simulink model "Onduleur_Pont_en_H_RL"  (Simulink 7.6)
settings: Solver=ode15s  StartTime=0.0  StopTime=10  RelTol=1e-3
InitFcn:
  | clc
  | R=1e3; C=2500e-3/(5*pi);%1e-3/(5*pi)
  | 
  | R1=1e3
  | R2=R1;
StopFcn:
  | if 0
  | clc
  | close all, clc
  | load U_Umoy_charge.mat
  | plot(x(1,:),x(2,:),x(1,:),x(3,:))
  | xlabel('temps')
  | title('Tension charge et sa valeur moyenne')
  | grid
  | 
  | load I_Imoy_charge.mat
  | figure
  | plot(y(1,:),y(2,:),y(1,:),y(3,:))
  | xlabel('temps')
  | title('Courant charge et sa valeur moyenne')
  | grid
  | 
  | delete *.mat
  | end
libraries: fl_lib x33, nesl_utility x16, powerlib x10, elec_lib x6

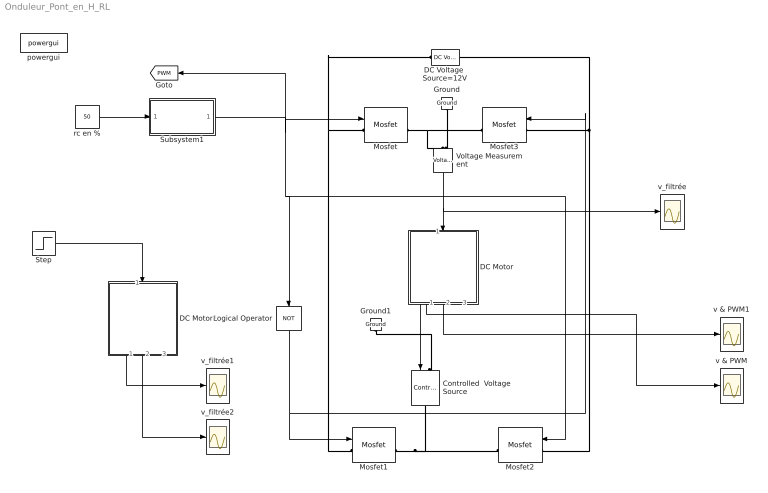
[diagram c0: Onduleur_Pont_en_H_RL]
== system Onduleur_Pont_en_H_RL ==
  Controlled  Voltage Source : powerlib/Electrical Sources/Controlled Voltage Source  DialogController=POWERSYS.PowerSysDialog  SystemSampleTime=-1  Initialize=on  Source_Type=AC  Amplitude=0  Phase=0  Frequency=0  Measurements=None
  DC Motor : Subsystem
  DC Motor1 : Subsystem
  DC Voltage  Source=12V : powerlib/Electrical Sources/DC Voltage Source  DialogController=POWERSYS.PowerSysDialog  SystemSampleTime=-1  Amplitude=12  Measurements=None
  Ground : powerlib/Elements/Ground  DialogController=POWERSYS.PowerSysDialog  PhysicalDomain=powersysdomain  SubClassName=unknown  LeftPortType=p1  RightPortType=p1  LConnTagsString=a
  Ground1 : powerlib/Elements/Ground  DialogController=POWERSYS.PowerSysDialog  PhysicalDomain=powersysdomain  SubClassName=unknown  LeftPortType=p1  RightPortType=p1  LConnTagsString=a
  Logical Operator : Logic  Operator=NOT  AllPortsSameDT=off  OutDataTypeStr=boolean
  Mosfet{,1..3} (4 alike) : powerlib/Power Electronics/Mosfet  DialogController=POWERSYS.PowerSysDialog  SystemSampleTime=-1  Ron=1e-6  Lon=0  Rd=0.001  Vfd=0  IC=0  Rs=1e8  Cs=inf  Measurements=on
  Step : Step  Time=2  After=12  SampleTime=0
  Subsystem1 : Subsystem
  Voltage Measurement : powerlib/Measurements/Voltage Measurement  DialogController=POWERSYS.PowerSysDialog  SystemSampleTime=-1  PhasorSimulation=off  OutputType=Complex  PSBequivalent=0
  powergui : powerlib/powergui  SystemSampleTime=-1  SimulationMode=Continuous  SampleTime=0  frequency=60  SPID=off  DisableSnubberDevices=off  DisableRonSwitches=off  DisableVfSwitches=off  SwTol=0  Interpol=off  frequencyindice=0  echomessages=off  HookPort=off  DisplayEquations=off  FunctionMessages=off  EnableUseOfTLC=off  x0status=blocks  RestoreLinks=warning  ResistiveCurrentMeasurement=off  Frange=[0:2:500]  Ylog=off  Xlog=on  ShowGrid=off  save=off  variable=ZData  ZoomFFT=on  StartTime=0.0  cycles=1  DisplayStyle=1  fundamental=60  FreqAxis=off  MaxFrequency=1000  frequencyindicesteady=1  RmsSteady=1  display=off  Ts=0  methode=off
  rc en % : Constant  Value=50
  v & PWM : Scope
  v & PWM1 : Scope
  v_filtrée : Scope
  v_filtrée1 : Scope
  v_filtrée2 : Scope
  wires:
  Subsystem1/1(PWM) -> Mosfet/1, Logical Operator/1, Mosfet2/1, [PWM]
  rc en %/1 -> Subsystem1/1(rc (%))
  Logical Operator/1 -> Mosfet1/1, Mosfet3/1
  Voltage Measurement/1 -> DC Motor/1(U+), v_filtrée/1
  DC Motor/3(U-) -> Controlled  Voltage Source/1
  DC Motor/1(w) -> v & PWM/1
  DC Motor/2(alpha) -> v & PWM1/1
  Step/1 -> DC Motor1/1(U+)
  DC Motor1/1(w) -> v_filtrée1/1
  DC Motor1/2(alpha) -> v_filtrée2/1
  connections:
  Mosfet1/RConn1 -- Mosfet2/RConn1 -- Controlled  Voltage Source/RConn1
  Mosfet/RConn1 -- Mosfet3/RConn1 -- Voltage Measurement/LConn1
  Mosfet1/LConn1 -- DC Voltage  Source=12V/LConn1 -- Mosfet/LConn1
  Mosfet2/LConn1 -- Mosfet3/LConn1 -- DC Voltage  Source=12V/RConn1
  Ground/LConn1 -- Voltage Measurement/LConn2
  Ground1/LConn1 -- Controlled  Voltage Source/LConn1

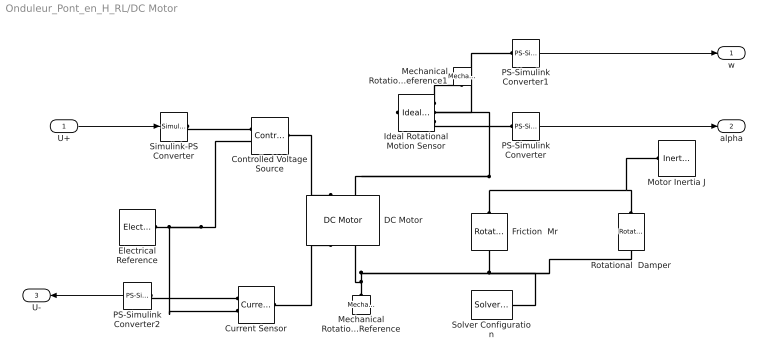
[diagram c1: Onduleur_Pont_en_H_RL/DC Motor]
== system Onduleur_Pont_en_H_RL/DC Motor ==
  U+ : Inport
  Controlled Voltage Source : fl_lib/Electrical/Electrical Sources/Controlled Voltage Source  DialogController=NetworkEngine.DynNeDlgSource  SystemSampleTime=-1  i_Log=off  v_Log=off  LocalVarNames=|i|v  LocalVarDescs=|i|v  LocalVarLogging=[0 0]
  Current Sensor : fl_lib/Electrical/Electrical Sensors/Current Sensor  DialogController=NetworkEngine.DynNeDlgSource  SystemSampleTime=-1  i1_Log=off  v1_Log=off  LocalVarNames=|i1|v1  LocalVarDescs=|i1|v1  LocalVarLogging=[0 0]
  DC Motor : elec_lib/Actuators & Drivers/Rotational Actuators/DC Motor  DialogController=NetworkEngine.DynNeDlgSource  SystemSampleTime=-1  parameterization=1  Ra=3.9 Ohm  La=1.2e-3 H  emf_or_torque=2  Kv=7.2e-5 V/rpm  Ki=10e-3 N*m/A  T_stall=2.4e-4 N*m  w_max=1.91e+4 rpm  w_rated=1.5e+4 rpm  P_rated=0.08 W  V_rated=1.5 V  J=0.01 g*cm^2  lam=1e-8 N*m/(rad/s)  speed0=0 rpm  current_Log=off  voltage_Log=off  power_Log=off  i2r_Log=off  torque_Log=off  speed_Log=off  LocalVarNames=|current|voltage|power|i2r|torque|speed  LocalVarDescs=|Current (A)|Voltage (V)|Power (W)|Electrical losses (W)|Torque (Nm)|Angular speed (rad/s)  LocalVarLogging=[0 0 0 0 0 0]
  Electrical Reference : fl_lib/Electrical/Electrical Elements/Electrical Reference  DialogController=NetworkEngine.DynNeDlgSource  SystemSampleTime=-1  i_Log=off  LocalVarNames=|i  LocalVarDescs=|i  LocalVarLogging=0
  Friction  Mr : fl_lib/Mechanical/Rotational Elements/Rotational Friction  DialogController=NetworkEngine.DynNeDlgSource  SystemSampleTime=-1  brkwy_trq=0.01e-3 N*m  Col_trq=0.01e-3 N*m  visc_coef=0.001e-3 N*m/(rad/s)  trans_coef=10 s/rad  vel_thr=0.1 rad/s  t_Log=off  w_Log=off  LocalVarNames=|friction_torque|rel_velocity|power  LocalVarDescs=|Friction torque (N*m)|Relative velocity (rad/s)|Power (W)  LocalVarLogging=[0 0 0]
  Ideal Rotational Motion Sensor : fl_lib/Mechanical/Mechanical Sensors/Ideal Rotational Motion Sensor  DialogController=NetworkEngine.DynNeDlgSource  SystemSampleTime=-1  offset=0 rad  w_Log=off  t_Log=off  phi_Log=off  LocalVarNames=|w|t|phi  LocalVarDescs=|w|t|phi  LocalVarLogging=[0 0 0]
  Mechanical Rotational Reference : fl_lib/Mechanical/Rotational Elements/Mechanical Rotational Reference  DialogController=NetworkEngine.DynNeDlgSource  SystemSampleTime=-1  t_Log=off  LocalVarNames=|t  LocalVarDescs=|t  LocalVarLogging=0
  Mechanical Rotational Reference1 : fl_lib/Mechanical/Rotational Elements/Mechanical Rotational Reference  DialogController=NetworkEngine.DynNeDlgSource  SystemSampleTime=-1  t_Log=off  LocalVarNames=|t  LocalVarDescs=|t  LocalVarLogging=0
  Motor Inertia J : fl_lib/Mechanical/Rotational Elements/Inertia  DialogController=NetworkEngine.DynNeDlgSource  SystemSampleTime=-1  inertia=0.01 g*cm^2  initial_velocity=0 rad/s  t_Log=off  LocalVarNames=|torque|velocity  LocalVarDescs=|Inertia torque (N*m)|Inertia absolute velocity (rad/s)  LocalVarLogging=[0 0]
  PS-Simulink Converter : nesl_utility/PS-Simulink Converter  DialogController=NetworkEngine.DynNeUtilDlgSource  SystemSampleTime=-1  PhysicalDomain=network_engine_domain  LeftPortType=input  RightPortType=output  SubClassName=ps_output  Unit=1  AffineConversion=off
  PS-Simulink Converter1 : nesl_utility/PS-Simulink Converter  DialogController=NetworkEngine.DynNeUtilDlgSource  SystemSampleTime=-1  PhysicalDomain=network_engine_domain  LeftPortType=input  RightPortType=output  SubClassName=ps_output  Unit=1  AffineConversion=off
  PS-Simulink Converter2 : nesl_utility/PS-Simulink Converter  DialogController=NetworkEngine.DynNeUtilDlgSource  SystemSampleTime=-1  PhysicalDomain=network_engine_domain  LeftPortType=input  RightPortType=output  SubClassName=ps_output  Unit=1  AffineConversion=off
  Rotational  Damper : fl_lib/Mechanical/Rotational Elements/Rotational Damper  DialogController=NetworkEngine.DynNeDlgSource  SystemSampleTime=-1  D=0.01 N*m/(rad/s)  t_Log=off  w_Log=off  LocalVarNames=|t|w  LocalVarDescs=|t|w  LocalVarLogging=[0 0]
  Simulink-PS Converter : nesl_utility/Simulink-PS Converter  DialogController=NetworkEngine.DynNeUtilDlgSource  SystemSampleTime=-1  PhysicalDomain=network_engine_domain  LeftPortType=input  RightPortType=output  SubClassName=ps_input  Unit=1  AffineConversion=off  InputFilterTimeConstant=.001  UdotUserProvided=0
  Solver Configuration : nesl_utility/Solver Configuration  DialogController=NetworkEngine.DynNeUtilDlgSource  SystemSampleTime=-1  PhysicalDomain=network_engine_domain  LeftPortType=input  RightPortType=generic  SubClassName=solver  Accelerate=off  Profile=off  ResidualTolerance=1e-9  MaxNonlinIter=3  MaxModeIter=2  DoFixedCost=off  UseLocalSampling=off  DoDC=off  LinearAlgebra=Sparse  LocalSolverSampleTime=.001  LocalSolverChoice=NE_BACKWARD_EULER_ADVANCER  UseLocalSolver=off
  w : Outport
  alpha : Outport  Port=2
  U- : Outport  Port=3
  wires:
  PS-Simulink Converter2/1 -> U-/1
  PS-Simulink Converter1/1 -> w/1
  PS-Simulink Converter/1 -> alpha/1
  U+/1 -> Simulink-PS Converter/1
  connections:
  PS-Simulink Converter2/LConn1 -- Current Sensor/RConn1
  Electrical Reference/LConn1 -- Current Sensor/RConn2 -- Controlled Voltage Source/RConn2
  Ideal Rotational Motion Sensor/RConn3 -- PS-Simulink Converter/LConn1
  Ideal Rotational Motion Sensor/RConn2 -- PS-Simulink Converter1/LConn1
  Ideal Rotational Motion Sensor/RConn1 -- Mechanical Rotational Reference1/LConn1
  Mechanical Rotational Reference/LConn1 -- DC Motor/RConn2 -- Friction  Mr/RConn1 -- Rotational  Damper/RConn1 -- Solver Configuration/RConn1
  Rotational  Damper/LConn1 -- Ideal Rotational Motion Sensor/LConn1 -- DC Motor/LConn2 -- Friction  Mr/LConn1 -- Motor Inertia J/LConn1
  Current Sensor/LConn1 -- DC Motor/RConn1
  Simulink-PS Converter/RConn1 -- Controlled Voltage Source/RConn1
  Controlled Voltage Source/LConn1 -- DC Motor/LConn1

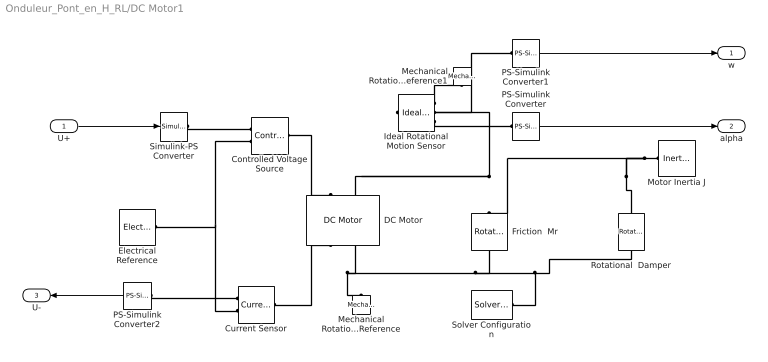
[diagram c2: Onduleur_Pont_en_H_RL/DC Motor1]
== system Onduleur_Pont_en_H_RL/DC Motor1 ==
  U+ : Inport
  Controlled Voltage Source : fl_lib/Electrical/Electrical Sources/Controlled Voltage Source  DialogController=NetworkEngine.DynNeDlgSource  SystemSampleTime=-1  i_Log=off  v_Log=off  LocalVarNames=|i|v  LocalVarDescs=|i|v  LocalVarLogging=[0 0]
  Current Sensor : fl_lib/Electrical/Electrical Sensors/Current Sensor  DialogController=NetworkEngine.DynNeDlgSource  SystemSampleTime=-1  i1_Log=off  v1_Log=off  LocalVarNames=|i1|v1  LocalVarDescs=|i1|v1  LocalVarLogging=[0 0]
  DC Motor : elec_lib/Actuators & Drivers/Rotational Actuators/DC Motor  DialogController=NetworkEngine.DynNeDlgSource  SystemSampleTime=-1  parameterization=1  Ra=3.9 Ohm  La=1.2e-3 H  emf_or_torque=2  Kv=7.2e-5 V/rpm  Ki=10e-3 N*m/A  T_stall=2.4e-4 N*m  w_max=1.91e+4 rpm  w_rated=1.5e+4 rpm  P_rated=0.08 W  V_rated=1.5 V  J=0.01 g*cm^2  lam=1e-8 N*m/(rad/s)  speed0=0 rpm  current_Log=off  voltage_Log=off  power_Log=off  i2r_Log=off  torque_Log=off  speed_Log=off  LocalVarNames=|current|voltage|power|i2r|torque|speed  LocalVarDescs=|Current (A)|Voltage (V)|Power (W)|Electrical losses (W)|Torque (Nm)|Angular speed (rad/s)  LocalVarLogging=[0 0 0 0 0 0]
  Electrical Reference : fl_lib/Electrical/Electrical Elements/Electrical Reference  DialogController=NetworkEngine.DynNeDlgSource  SystemSampleTime=-1  i_Log=off  LocalVarNames=|i  LocalVarDescs=|i  LocalVarLogging=0
  Friction  Mr : fl_lib/Mechanical/Rotational Elements/Rotational Friction  DialogController=NetworkEngine.DynNeDlgSource  SystemSampleTime=-1  brkwy_trq=0.001 N*m  Col_trq=0.001 N*m  visc_coef=0.001 N*m/(rad/s)  trans_coef=10 s/rad  vel_thr=0.1 rad/s  t_Log=off  w_Log=off  LocalVarNames=|friction_torque|rel_velocity|power  LocalVarDescs=|Friction torque (N*m)|Relative velocity (rad/s)|Power (W)  LocalVarLogging=[0 0 0]
  Ideal Rotational Motion Sensor : fl_lib/Mechanical/Mechanical Sensors/Ideal Rotational Motion Sensor  DialogController=NetworkEngine.DynNeDlgSource  SystemSampleTime=-1  offset=0 rad  w_Log=off  t_Log=off  phi_Log=off  LocalVarNames=|w|t|phi  LocalVarDescs=|w|t|phi  LocalVarLogging=[0 0 0]
  Mechanical Rotational Reference : fl_lib/Mechanical/Rotational Elements/Mechanical Rotational Reference  DialogController=NetworkEngine.DynNeDlgSource  SystemSampleTime=-1  t_Log=off  LocalVarNames=|t  LocalVarDescs=|t  LocalVarLogging=0
  Mechanical Rotational Reference1 : fl_lib/Mechanical/Rotational Elements/Mechanical Rotational Reference  DialogController=NetworkEngine.DynNeDlgSource  SystemSampleTime=-1  t_Log=off  LocalVarNames=|t  LocalVarDescs=|t  LocalVarLogging=0
  Motor Inertia J : fl_lib/Mechanical/Rotational Elements/Inertia  DialogController=NetworkEngine.DynNeDlgSource  SystemSampleTime=-1  inertia=0.1 g*cm^2  initial_velocity=0 rad/s  t_Log=off  LocalVarNames=|torque|velocity  LocalVarDescs=|Inertia torque (N*m)|Inertia absolute velocity (rad/s)  LocalVarLogging=[0 0]
  PS-Simulink Converter : nesl_utility/PS-Simulink Converter  DialogController=NetworkEngine.DynNeUtilDlgSource  SystemSampleTime=-1  PhysicalDomain=network_engine_domain  LeftPortType=input  RightPortType=output  SubClassName=ps_output  Unit=1  AffineConversion=off
  PS-Simulink Converter1 : nesl_utility/PS-Simulink Converter  DialogController=NetworkEngine.DynNeUtilDlgSource  SystemSampleTime=-1  PhysicalDomain=network_engine_domain  LeftPortType=input  RightPortType=output  SubClassName=ps_output  Unit=1  AffineConversion=off
  PS-Simulink Converter2 : nesl_utility/PS-Simulink Converter  DialogController=NetworkEngine.DynNeUtilDlgSource  SystemSampleTime=-1  PhysicalDomain=network_engine_domain  LeftPortType=input  RightPortType=output  SubClassName=ps_output  Unit=1  AffineConversion=off
  Rotational  Damper : fl_lib/Mechanical/Rotational Elements/Rotational Damper  DialogController=NetworkEngine.DynNeDlgSource  SystemSampleTime=-1  D=0.01 N*m/(rad/s)  t_Log=off  w_Log=off  LocalVarNames=|t|w  LocalVarDescs=|t|w  LocalVarLogging=[0 0]
  Simulink-PS Converter : nesl_utility/Simulink-PS Converter  DialogController=NetworkEngine.DynNeUtilDlgSource  SystemSampleTime=-1  PhysicalDomain=network_engine_domain  LeftPortType=input  RightPortType=output  SubClassName=ps_input  Unit=1  AffineConversion=off  InputFilterTimeConstant=.001  UdotUserProvided=0
  Solver Configuration : nesl_utility/Solver Configuration  DialogController=NetworkEngine.DynNeUtilDlgSource  SystemSampleTime=-1  PhysicalDomain=network_engine_domain  LeftPortType=input  RightPortType=generic  SubClassName=solver  Accelerate=off  Profile=off  ResidualTolerance=1e-9  MaxNonlinIter=3  MaxModeIter=2  DoFixedCost=off  UseLocalSampling=off  DoDC=off  LinearAlgebra=Sparse  LocalSolverSampleTime=.001  LocalSolverChoice=NE_BACKWARD_EULER_ADVANCER  UseLocalSolver=off
  w : Outport
  alpha : Outport  Port=2
  U- : Outport  Port=3
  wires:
  U+/1 -> Simulink-PS Converter/1
  PS-Simulink Converter/1 -> alpha/1
  PS-Simulink Converter1/1 -> w/1
  PS-Simulink Converter2/1 -> U-/1
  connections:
  Controlled Voltage Source/LConn1 -- DC Motor/LConn1
  Simulink-PS Converter/RConn1 -- Controlled Voltage Source/RConn1
  Current Sensor/LConn1 -- DC Motor/RConn1
  Motor Inertia J/LConn1 -- Friction  Mr/LConn1 -- DC Motor/LConn2 -- Ideal Rotational Motion Sensor/LConn1 -- Rotational  Damper/LConn1
  Solver Configuration/RConn1 -- Rotational  Damper/RConn1 -- Friction  Mr/RConn1 -- DC Motor/RConn2 -- Mechanical Rotational Reference/LConn1
  Ideal Rotational Motion Sensor/RConn1 -- Mechanical Rotational Reference1/LConn1
  Ideal Rotational Motion Sensor/RConn2 -- PS-Simulink Converter1/LConn1
  Ideal Rotational Motion Sensor/RConn3 -- PS-Simulink Converter/LConn1
  Controlled Voltage Source/RConn2 -- Current Sensor/RConn2 -- Electrical Reference/LConn1
  PS-Simulink Converter2/LConn1 -- Current Sensor/RConn1

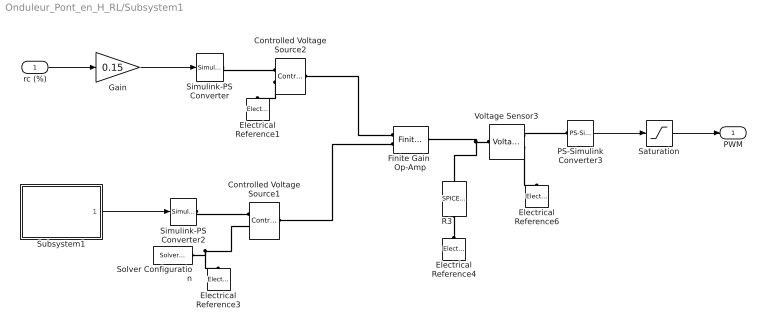
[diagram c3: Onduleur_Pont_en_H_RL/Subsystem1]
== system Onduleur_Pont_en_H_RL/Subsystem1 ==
  rc (%) : Inport
  Controlled Voltage Source1 : fl_lib/Electrical/Electrical Sources/Controlled Voltage Source  DialogController=NetworkEngine.DynNeDlgSource  SystemSampleTime=-1  i_Log=off  v_Log=off  LocalVarNames=|current|voltage|power  LocalVarDescs=|Current (A)|Voltage (V)|Power (W)  LocalVarLogging=[0 0 0]
  Controlled Voltage Source2 : fl_lib/Electrical/Electrical Sources/Controlled Voltage Source  DialogController=NetworkEngine.DynNeDlgSource  SystemSampleTime=-1  i_Log=off  v_Log=off  LocalVarNames=|current|voltage|power  LocalVarDescs=|Current (A)|Voltage (V)|Power (W)  LocalVarLogging=[0 0 0]
  Electrical Reference{1,3..4,6} (4 alike) : fl_lib/Electrical/Electrical Elements/Electrical Reference  DialogController=NetworkEngine.DynNeDlgSource  SystemSampleTime=-1  i_Log=off  LocalVarNames=|i  LocalVarDescs=|i  LocalVarLogging=[]
  Finite Gain  Op-Amp : elec_lib/Integrated Circuits/Finite Gain Op-Amp  DialogController=NetworkEngine.DynNeDlgSource  SystemSampleTime=-1  A=1000  Rin=1e+06 Ohm  Rout=100 Ohm  Vmin=-12 V  Vmax=12 V  LocalVarNames=|power  LocalVarDescs=|Dissipated power (W)  LocalVarLogging=0
  Gain : Gain  Gain=0.15
  PS-Simulink Converter3 : nesl_utility/PS-Simulink Converter  DialogController=NetworkEngine.DynNeUtilDlgSource  SystemSampleTime=-1  PhysicalDomain=network_engine_domain  LeftPortType=input  RightPortType=output  SubClassName=ps_output  Unit=1  AffineConversion=off
  R3 : elec_lib/Additional Components/SPICE-Compatible Components/Passive Devices/SPICE Resistor  DialogController=NetworkEngine.DynNeDlgSource  SystemSampleTime=-1  SCALE=1  R_param=1  R=10e3 Ohm  RSH=0 Ohm  LENGTH=1e-06 m  WIDTH=1e-06 m  NARROW=0 m  T_param=1  TC1=0 1/K  TC2=0 1/K^2  TOFFSET=0 K  TFIXED=300.15 K  TMEAS=300.15 K  LocalVarLogging=[]
  Saturation : Saturate  UpperLimit=1  LowerLimit=0
  Simulink-PS Converter : nesl_utility/Simulink-PS Converter  DialogController=NetworkEngine.DynNeUtilDlgSource  SystemSampleTime=-1  PhysicalDomain=network_engine_domain  LeftPortType=input  RightPortType=output  SubClassName=ps_input  Unit=1  AffineConversion=off  InputFilterTimeConstant=.001  UdotUserProvided=0
  Simulink-PS Converter2 : nesl_utility/Simulink-PS Converter  DialogController=NetworkEngine.DynNeUtilDlgSource  SystemSampleTime=-1  PhysicalDomain=network_engine_domain  LeftPortType=input  RightPortType=output  SubClassName=ps_input  Unit=1  AffineConversion=off  InputFilterTimeConstant=.001  UdotUserProvided=0
  Solver Configuration : nesl_utility/Solver Configuration  DialogController=NetworkEngine.DynNeUtilDlgSource  SystemSampleTime=-1  PhysicalDomain=network_engine_domain  LeftPortType=input  RightPortType=generic  SubClassName=solver  Accelerate=off  Profile=off  ResidualTolerance=1e-12  MaxNonlinIter=12  MaxModeIter=2  DoFixedCost=on  UseLocalSampling=off  DoDC=off  LinearAlgebra=Sparse  LocalSolverSampleTime=.001  LocalSolverChoice=NE_BACKWARD_EULER_ADVANCER  UseLocalSolver=off
  Subsystem1 : Subsystem
  Voltage Sensor3 : fl_lib/Electrical/Electrical Sensors/Voltage Sensor  DialogController=NetworkEngine.DynNeDlgSource  SystemSampleTime=-1  i1_Log=off  v1_Log=off  LocalVarNames=|i1|v1  LocalVarDescs=|i1|v1  LocalVarLogging=[]
  PWM : Outport
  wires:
  Gain/1 -> Simulink-PS Converter/1
  Saturation/1 -> PWM/1
  PS-Simulink Converter3/1 -> Saturation/1
  rc (%)/1 -> Gain/1
  Subsystem1/1(tri) -> Simulink-PS Converter2/1
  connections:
  Voltage Sensor3/RConn1 -- PS-Simulink Converter3/LConn1
  Voltage Sensor3/LConn1 -- R3/RConn1 -- Finite Gain  Op-Amp/RConn1
  Voltage Sensor3/RConn2 -- Electrical Reference6/LConn1
  Electrical Reference4/LConn1 -- R3/LConn1
  Controlled Voltage Source2/RConn2 -- Electrical Reference1/LConn1
  Simulink-PS Converter/RConn1 -- Controlled Voltage Source2/RConn1
  Finite Gain  Op-Amp/LConn1 -- Controlled Voltage Source2/LConn1
  Solver Configuration/RConn1 -- Electrical Reference3/LConn1 -- Controlled Voltage Source1/RConn2
  Simulink-PS Converter2/RConn1 -- Controlled Voltage Source1/RConn1
  Controlled Voltage Source1/LConn1 -- Finite Gain  Op-Amp/LConn2

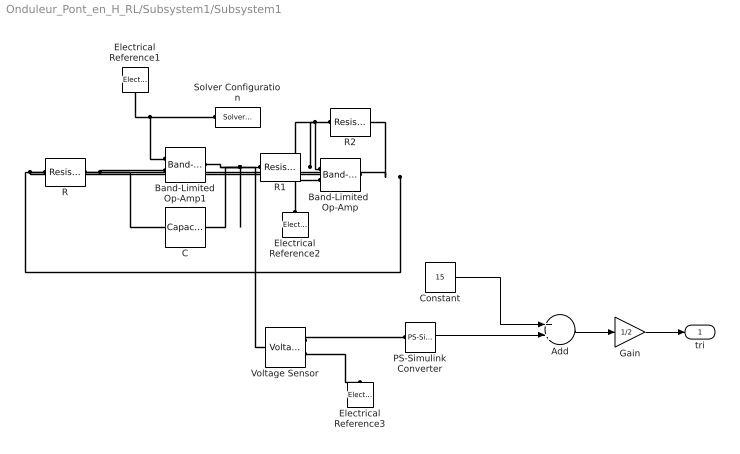
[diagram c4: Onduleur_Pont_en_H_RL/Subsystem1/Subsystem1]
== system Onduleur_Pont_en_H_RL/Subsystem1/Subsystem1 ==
  Add : Sum
  Band-Limited  Op-Amp : elec_lib/Integrated Circuits/Band-Limited Op-Amp  DialogController=NetworkEngine.DynNeDlgSource  SystemSampleTime=-1  A=1000  Rin=1e+06 Ohm  Rout=100 Ohm  Vmin=-15 V  Vmax=15 V  Vdotmax=1000 V/s  f=1e+05 Hz  V0=0 V  LocalVarNames=|power  LocalVarDescs=|Dissipated power (W)  LocalVarLogging=0
  Band-Limited Op-Amp1 : elec_lib/Integrated Circuits/Band-Limited Op-Amp  DialogController=NetworkEngine.DynNeDlgSource  SystemSampleTime=-1  A=1000  Rin=1e+06 Ohm  Rout=100 Ohm  Vmin=-15 V  Vmax=15 V  Vdotmax=1000 V/s  f=1e+05 Hz  V0=0 V  LocalVarNames=|power  LocalVarDescs=|Dissipated power (W)  LocalVarLogging=0
  C : fl_lib/Electrical/Electrical Elements/Capacitor  DialogController=NetworkEngine.DynNeDlgSource  SystemSampleTime=-1  c=0.5e-4 F  v0=0.1 V  r=1e-6 Ohm  g=0 1/Ohm  i_Log=off  v_Log=off  vc_Log=off  LocalVarNames=|current|voltage|power  LocalVarDescs=|Capacitor current (A)|Voltage across capacitor (V)|Power (W)  LocalVarLogging=[0 0 0]
  Constant : Constant  Value=15
  Electrical Reference1 : fl_lib/Electrical/Electrical Elements/Electrical Reference  DialogController=NetworkEngine.DynNeDlgSource  SystemSampleTime=-1  i_Log=off  LocalVarNames=|i  LocalVarDescs=|i  LocalVarLogging=[]
  Electrical Reference2 : fl_lib/Electrical/Electrical Elements/Electrical Reference  DialogController=NetworkEngine.DynNeDlgSource  SystemSampleTime=-1  i_Log=off  LocalVarNames=|i  LocalVarDescs=|i  LocalVarLogging=[]
  Electrical Reference3 : fl_lib/Electrical/Electrical Elements/Electrical Reference  DialogController=NetworkEngine.DynNeDlgSource  SystemSampleTime=-1  i_Log=off  LocalVarNames=|i  LocalVarDescs=|i  LocalVarLogging=[]
  Gain : Gain  Gain=1/2
  PS-Simulink Converter : nesl_utility/PS-Simulink Converter  DialogController=NetworkEngine.DynNeUtilDlgSource  SystemSampleTime=-1  PhysicalDomain=network_engine_domain  LeftPortType=input  RightPortType=output  SubClassName=ps_output  Unit=1  AffineConversion=off
  R : fl_lib/Electrical/Electrical Elements/Resistor  DialogController=NetworkEngine.DynNeDlgSource  SystemSampleTime=-1  R=1000 Ohm  i_Log=off  v_Log=off  LocalVarNames=|current|voltage|power  LocalVarDescs=|Resistor current (A)|Voltage across resistor (V)|Power (W)  LocalVarLogging=[0 0 0]
  R1 : fl_lib/Electrical/Electrical Elements/Resistor  DialogController=NetworkEngine.DynNeDlgSource  SystemSampleTime=-1  R=10e3 Ohm  i_Log=off  v_Log=off  LocalVarNames=|current|voltage|power  LocalVarDescs=|Resistor current (A)|Voltage across resistor (V)|Power (W)  LocalVarLogging=[0 0 0]
  R2 : fl_lib/Electrical/Electrical Elements/Resistor  DialogController=NetworkEngine.DynNeDlgSource  SystemSampleTime=-1  R=10e3 Ohm  i_Log=off  v_Log=off  LocalVarNames=|current|voltage|power  LocalVarDescs=|Resistor current (A)|Voltage across resistor (V)|Power (W)  LocalVarLogging=[0 0 0]
  Solver Configuration : nesl_utility/Solver Configuration  DialogController=NetworkEngine.DynNeUtilDlgSource  SystemSampleTime=-1  PhysicalDomain=network_engine_domain  LeftPortType=input  RightPortType=generic  SubClassName=solver  Accelerate=off  Profile=off  ResidualTolerance=1e-9  MaxNonlinIter=12  MaxModeIter=2  DoFixedCost=off  UseLocalSampling=off  DoDC=off  LinearAlgebra=Sparse  LocalSolverSampleTime=.001  LocalSolverChoice=NE_BACKWARD_EULER_ADVANCER  UseLocalSolver=off
  Voltage Sensor : fl_lib/Electrical/Electrical Sensors/Voltage Sensor  DialogController=NetworkEngine.DynNeDlgSource  SystemSampleTime=-1  i1_Log=off  v1_Log=off  LocalVarNames=|i1|v1  LocalVarDescs=|i1|v1  LocalVarLogging=[]
  tri : Outport
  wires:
  PS-Simulink Converter/1 -> Add/2
  Constant/1 -> Add/1
  Add/1 -> Gain/1
  Gain/1 -> tri/1
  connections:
  Voltage Sensor/RConn1 -- PS-Simulink Converter/LConn1
  Band-Limited Op-Amp1/RConn1 -- R1/LConn1 -- C/RConn1 -- Voltage Sensor/LConn1
  R/RConn1 -- C/LConn1 -- Band-Limited Op-Amp1/LConn2
  Solver Configuration/RConn1 -- Band-Limited Op-Amp1/LConn1 -- Electrical Reference1/LConn1
  R/LConn1 -- Band-Limited  Op-Amp/RConn1 -- R2/RConn1
  Electrical Reference2/LConn1 -- Band-Limited  Op-Amp/LConn2
  R2/LConn1 -- Band-Limited  Op-Amp/LConn1 -- R1/RConn1
  Voltage Sensor/RConn2 -- Electrical Reference3/LConn1
